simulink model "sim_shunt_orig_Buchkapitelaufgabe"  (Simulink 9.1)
settings: Solver=ode23s  StartTime=0.0  StopTime=4000  RelTol=1e-8  EnableMultiTasking=on
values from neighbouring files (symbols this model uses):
  Bauchdruck = 0    [InitVentil_Buchkapitel.m]
  HydrHoehe = sin(Liegewinkel)*l_Schlauch*73.55    [InitVentil_Buchkapitel.m]
  ICP_n = 0.9330    (= 0.933)    [InitVentil_Buchkapitel.m]
  ICP_shift = 9*sin(Liegewinkel*2 + pi/2)+5 - 14    [InitVentil_Buchkapitel.m]
  R_hyd = 128*eta_Liquor*l_Schlauch/(pi*d_Schlauch^4)*Umrechnungsfaktor    (= 68180382716.6)    [InitVentil_Buchkapitel.m]
  ventil_oeffn = 7    [InitVentil_Buchkapitel.m]
undefined symbols (not defined in the file or in its folder): ABP_n, alph, alphco2, G_vor, h_01, h_02, h_0_ven, ini1_reg, ini2_reg, K_e1, K_e2, K_e_ven, K_G1, K_G2, K_G_ven, k_prod, k_res, K_v1, K_v2, K_v_ven, n_m1, n_m2, O2_verb, p1_n, Pco2_AB, PCO2_soll, Po2_ab, PO2_blut, PO2_soll, r1_100, r2_100, r2_n, r_01, r_02, r_0_ven, r_m1, r_m2, r_t1, r_t2, rv_100, sigma_01, sigma_02, sigma_0_ven, sigma_0_visk_1, sigma_0_visk_2, sigma_koll1, sigma_koll2, sigma_koll_ven, sigma_m01, sigma_m02, V, V1_n, V2_n, V_ven_0, VBPss_n
libraries: neural x36, simulink_extras x3, simulink x1
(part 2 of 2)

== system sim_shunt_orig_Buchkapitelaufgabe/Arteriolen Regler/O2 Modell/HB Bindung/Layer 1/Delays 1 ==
  "p{1}" : Inport  PortDimensions=1
  mux : Mux  Inputs=1
  "pd{1,1}" : Outport
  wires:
  "p{1}"/1 -> mux/1
  mux/1 -> "pd{1,1}"/1

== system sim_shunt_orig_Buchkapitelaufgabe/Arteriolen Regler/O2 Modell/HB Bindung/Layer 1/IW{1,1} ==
  "pd{1,1}" : Inport  PortDimensions=1
  "IW{1,1}(1,:)'" : Constant  Value=-0.064707731186413736
  "IW{1,1}(2,:)'" : Constant  Value=-0.14661098203804576
  Mux : Mux  Inputs=2
  dotprod1 : neural/Weight Functions/dotprod
  dotprod2 : neural/Weight Functions/dotprod
  "iz{1,1}" : Outport
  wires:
  "IW{1,1}(1,:)'"/1 -> dotprod1/1
  dotprod1/1 -> Mux/1
  "IW{1,1}(2,:)'"/1 -> dotprod2/1
  "pd{1,1}"/1 -> dotprod1/2, dotprod2/2
  dotprod2/1 -> Mux/2
  Mux/1 -> "iz{1,1}"/1

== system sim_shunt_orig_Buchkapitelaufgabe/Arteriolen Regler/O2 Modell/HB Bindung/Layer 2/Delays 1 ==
  "p{2}" : Inport  PortDimensions=2
  mux : Mux  Inputs=1
  "pd{2,1}" : Outport
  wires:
  "p{2}"/1 -> mux/1
  mux/1 -> "pd{2,1}"/1

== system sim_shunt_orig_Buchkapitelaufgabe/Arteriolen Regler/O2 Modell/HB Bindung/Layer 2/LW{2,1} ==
  "ad{2,1}" : Inport  PortDimensions=2
  "IW{2,1}(1,:)'" : Constant  Value=[-21.951961087859253;6.8232958826842776]
  Mux : Mux  Inputs=1
  dotprod1 : neural/Weight Functions/dotprod
  "lz{2,1}" : Outport
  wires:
  "IW{2,1}(1,:)'"/1 -> dotprod1/1
  "ad{2,1}"/1 -> dotprod1/2
  dotprod1/1 -> Mux/1
  Mux/1 -> "lz{2,1}"/1

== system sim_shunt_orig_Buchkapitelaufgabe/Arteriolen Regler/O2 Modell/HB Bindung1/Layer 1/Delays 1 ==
  "p{1}" : Inport  PortDimensions=1
  mux : Mux  Inputs=1
  "pd{1,1}" : Outport
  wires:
  mux/1 -> "pd{1,1}"/1
  "p{1}"/1 -> mux/1

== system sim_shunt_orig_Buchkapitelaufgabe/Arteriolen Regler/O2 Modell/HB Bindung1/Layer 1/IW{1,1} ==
  "pd{1,1}" : Inport  PortDimensions=1
  "IW{1,1}(1,:)'" : Constant  Value=-0.064707731186413736
  "IW{1,1}(2,:)'" : Constant  Value=-0.14661098203804576
  Mux : Mux  Inputs=2
  dotprod1 : neural/Weight Functions/dotprod
  dotprod2 : neural/Weight Functions/dotprod
  "iz{1,1}" : Outport
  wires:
  Mux/1 -> "iz{1,1}"/1
  dotprod2/1 -> Mux/2
  "pd{1,1}"/1 -> dotprod2/2, dotprod1/2
  "IW{1,1}(2,:)'"/1 -> dotprod2/1
  dotprod1/1 -> Mux/1
  "IW{1,1}(1,:)'"/1 -> dotprod1/1

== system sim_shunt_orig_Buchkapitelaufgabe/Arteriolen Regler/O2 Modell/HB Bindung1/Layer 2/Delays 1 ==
  "p{2}" : Inport  PortDimensions=2
  mux : Mux  Inputs=1
  "pd{2,1}" : Outport
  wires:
  mux/1 -> "pd{2,1}"/1
  "p{2}"/1 -> mux/1

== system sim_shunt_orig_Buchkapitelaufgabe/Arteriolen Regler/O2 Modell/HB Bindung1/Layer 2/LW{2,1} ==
  "ad{2,1}" : Inport  PortDimensions=2
  "IW{2,1}(1,:)'" : Constant  Value=[-21.951961087859253;6.8232958826842776]
  Mux : Mux  Inputs=1
  dotprod1 : neural/Weight Functions/dotprod
  "lz{2,1}" : Outport
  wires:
  Mux/1 -> "lz{2,1}"/1
  dotprod1/1 -> Mux/1
  "ad{2,1}"/1 -> dotprod1/2
  "IW{2,1}(1,:)'"/1 -> dotprod1/1

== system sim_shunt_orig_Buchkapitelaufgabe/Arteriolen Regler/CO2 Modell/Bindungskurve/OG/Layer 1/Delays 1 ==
  "p{1}" : Inport  PortDimensions=1
  mux : Mux  Inputs=1
  "pd{1,1}" : Outport
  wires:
  mux/1 -> "pd{1,1}"/1
  "p{1}"/1 -> mux/1

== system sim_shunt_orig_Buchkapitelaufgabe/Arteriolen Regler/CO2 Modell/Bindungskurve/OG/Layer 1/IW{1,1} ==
  "pd{1,1}" : Inport  PortDimensions=1
  "IW{1,1}(1,:)'" : Constant  Value=0.39084037748549827
  "IW{1,1}(2,:)'" : Constant  Value=0.022370352278219353
  "IW{1,1}(3,:)'" : Constant  Value=0.19403608090506319
  Mux : Mux  Inputs=3
  dotprod1 : neural/Weight Functions/dotprod
  dotprod2 : neural/Weight Functions/dotprod
  dotprod3 : neural/Weight Functions/dotprod
  "iz{1,1}" : Outport
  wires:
  Mux/1 -> "iz{1,1}"/1
  dotprod3/1 -> Mux/3
  "IW{1,1}(3,:)'"/1 -> dotprod3/1
  dotprod2/1 -> Mux/2
  "pd{1,1}"/1 -> dotprod3/2, dotprod2/2, dotprod1/2
  "IW{1,1}(2,:)'"/1 -> dotprod2/1
  dotprod1/1 -> Mux/1
  "IW{1,1}(1,:)'"/1 -> dotprod1/1

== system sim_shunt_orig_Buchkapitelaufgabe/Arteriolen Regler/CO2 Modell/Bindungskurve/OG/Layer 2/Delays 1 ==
  "p{2}" : Inport  PortDimensions=3
  mux : Mux  Inputs=1
  "pd{2,1}" : Outport
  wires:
  mux/1 -> "pd{2,1}"/1
  "p{2}"/1 -> mux/1

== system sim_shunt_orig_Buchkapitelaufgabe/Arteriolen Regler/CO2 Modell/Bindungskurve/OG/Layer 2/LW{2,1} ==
  "ad{2,1}" : Inport  PortDimensions=3
  "IW{2,1}(1,:)'" : Constant  Value=[-34.807144004972457;79.560951131325595;50.241573431449858]
  Mux : Mux  Inputs=1
  dotprod1 : neural/Weight Functions/dotprod
  "lz{2,1}" : Outport
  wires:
  Mux/1 -> "lz{2,1}"/1
  dotprod1/1 -> Mux/1
  "ad{2,1}"/1 -> dotprod1/2
  "IW{2,1}(1,:)'"/1 -> dotprod1/1

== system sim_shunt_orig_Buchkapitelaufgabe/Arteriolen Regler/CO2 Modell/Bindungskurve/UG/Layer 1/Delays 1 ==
  "p{1}" : Inport  PortDimensions=1
  mux : Mux  Inputs=1
  "pd{1,1}" : Outport
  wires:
  mux/1 -> "pd{1,1}"/1
  "p{1}"/1 -> mux/1

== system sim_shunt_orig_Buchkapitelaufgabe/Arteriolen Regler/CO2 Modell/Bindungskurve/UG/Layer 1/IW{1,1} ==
  "pd{1,1}" : Inport  PortDimensions=1
  "IW{1,1}(1,:)'" : Constant  Value=-0.056170689932274573
  "IW{1,1}(2,:)'" : Constant  Value=0.050617741606017563
  "IW{1,1}(3,:)'" : Constant  Value=0.59403476334946692
  Mux : Mux  Inputs=3
  dotprod1 : neural/Weight Functions/dotprod
  dotprod2 : neural/Weight Functions/dotprod
  dotprod3 : neural/Weight Functions/dotprod
  "iz{1,1}" : Outport
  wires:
  Mux/1 -> "iz{1,1}"/1
  dotprod3/1 -> Mux/3
  "IW{1,1}(3,:)'"/1 -> dotprod3/1
  dotprod2/1 -> Mux/2
  "pd{1,1}"/1 -> dotprod3/2, dotprod2/2, dotprod1/2
  "IW{1,1}(2,:)'"/1 -> dotprod2/1
  dotprod1/1 -> Mux/1
  "IW{1,1}(1,:)'"/1 -> dotprod1/1

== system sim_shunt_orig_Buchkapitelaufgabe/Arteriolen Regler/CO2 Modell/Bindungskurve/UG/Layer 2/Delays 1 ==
  "p{2}" : Inport  PortDimensions=3
  mux : Mux  Inputs=1
  "pd{2,1}" : Outport
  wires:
  mux/1 -> "pd{2,1}"/1
  "p{2}"/1 -> mux/1

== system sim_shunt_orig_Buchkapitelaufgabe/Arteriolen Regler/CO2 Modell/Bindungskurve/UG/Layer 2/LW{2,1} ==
  "ad{2,1}" : Inport  PortDimensions=3
  "IW{2,1}(1,:)'" : Constant  Value=[-73.411517044567987;10.445427355877589;30.151834894692133]
  Mux : Mux  Inputs=1
  dotprod1 : neural/Weight Functions/dotprod
  "lz{2,1}" : Outport
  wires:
  Mux/1 -> "lz{2,1}"/1
  dotprod1/1 -> Mux/1
  "ad{2,1}"/1 -> dotprod1/2
  "IW{2,1}(1,:)'"/1 -> dotprod1/1

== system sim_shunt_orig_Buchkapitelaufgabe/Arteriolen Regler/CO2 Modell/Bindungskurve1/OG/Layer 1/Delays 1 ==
  "p{1}" : Inport  PortDimensions=1
  mux : Mux  Inputs=1
  "pd{1,1}" : Outport
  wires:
  "p{1}"/1 -> mux/1
  mux/1 -> "pd{1,1}"/1

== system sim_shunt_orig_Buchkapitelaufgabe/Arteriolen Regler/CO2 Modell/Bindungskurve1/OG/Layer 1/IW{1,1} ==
  "pd{1,1}" : Inport  PortDimensions=1
  "IW{1,1}(1,:)'" : Constant  Value=0.39084037748549827
  "IW{1,1}(2,:)'" : Constant  Value=0.022370352278219353
  "IW{1,1}(3,:)'" : Constant  Value=0.19403608090506319
  Mux : Mux  Inputs=3
  dotprod1 : neural/Weight Functions/dotprod
  dotprod2 : neural/Weight Functions/dotprod
  dotprod3 : neural/Weight Functions/dotprod
  "iz{1,1}" : Outport
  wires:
  "IW{1,1}(1,:)'"/1 -> dotprod1/1
  dotprod1/1 -> Mux/1
  "IW{1,1}(2,:)'"/1 -> dotprod2/1
  "pd{1,1}"/1 -> dotprod1/2, dotprod2/2, dotprod3/2
  dotprod2/1 -> Mux/2
  "IW{1,1}(3,:)'"/1 -> dotprod3/1
  dotprod3/1 -> Mux/3
  Mux/1 -> "iz{1,1}"/1

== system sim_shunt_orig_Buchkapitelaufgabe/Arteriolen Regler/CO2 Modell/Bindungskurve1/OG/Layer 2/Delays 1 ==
  "p{2}" : Inport  PortDimensions=3
  mux : Mux  Inputs=1
  "pd{2,1}" : Outport
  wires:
  "p{2}"/1 -> mux/1
  mux/1 -> "pd{2,1}"/1

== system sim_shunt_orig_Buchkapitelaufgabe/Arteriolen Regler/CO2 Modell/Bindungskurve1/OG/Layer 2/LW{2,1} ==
  "ad{2,1}" : Inport  PortDimensions=3
  "IW{2,1}(1,:)'" : Constant  Value=[-34.807144004972457;79.560951131325595;50.241573431449858]
  Mux : Mux  Inputs=1
  dotprod1 : neural/Weight Functions/dotprod
  "lz{2,1}" : Outport
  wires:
  "IW{2,1}(1,:)'"/1 -> dotprod1/1
  "ad{2,1}"/1 -> dotprod1/2
  dotprod1/1 -> Mux/1
  Mux/1 -> "lz{2,1}"/1

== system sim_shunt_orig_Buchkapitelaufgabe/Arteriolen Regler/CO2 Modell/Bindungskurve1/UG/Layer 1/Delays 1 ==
  "p{1}" : Inport  PortDimensions=1
  mux : Mux  Inputs=1
  "pd{1,1}" : Outport
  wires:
  "p{1}"/1 -> mux/1
  mux/1 -> "pd{1,1}"/1

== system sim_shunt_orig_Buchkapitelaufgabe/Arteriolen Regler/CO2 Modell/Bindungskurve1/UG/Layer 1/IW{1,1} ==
  "pd{1,1}" : Inport  PortDimensions=1
  "IW{1,1}(1,:)'" : Constant  Value=-0.056170689932274573
  "IW{1,1}(2,:)'" : Constant  Value=0.050617741606017563
  "IW{1,1}(3,:)'" : Constant  Value=0.59403476334946692
  Mux : Mux  Inputs=3
  dotprod1 : neural/Weight Functions/dotprod
  dotprod2 : neural/Weight Functions/dotprod
  dotprod3 : neural/Weight Functions/dotprod
  "iz{1,1}" : Outport
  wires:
  "IW{1,1}(1,:)'"/1 -> dotprod1/1
  dotprod1/1 -> Mux/1
  "IW{1,1}(2,:)'"/1 -> dotprod2/1
  "pd{1,1}"/1 -> dotprod1/2, dotprod2/2, dotprod3/2
  dotprod2/1 -> Mux/2
  "IW{1,1}(3,:)'"/1 -> dotprod3/1
  dotprod3/1 -> Mux/3
  Mux/1 -> "iz{1,1}"/1

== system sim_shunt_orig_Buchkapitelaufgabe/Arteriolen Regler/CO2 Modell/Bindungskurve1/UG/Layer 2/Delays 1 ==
  "p{2}" : Inport  PortDimensions=3
  mux : Mux  Inputs=1
  "pd{2,1}" : Outport
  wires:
  "p{2}"/1 -> mux/1
  mux/1 -> "pd{2,1}"/1

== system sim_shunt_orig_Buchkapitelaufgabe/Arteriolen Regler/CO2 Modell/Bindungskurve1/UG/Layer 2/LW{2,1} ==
  "ad{2,1}" : Inport  PortDimensions=3
  "IW{2,1}(1,:)'" : Constant  Value=[-73.411517044567987;10.445427355877589;30.151834894692133]
  Mux : Mux  Inputs=1
  dotprod1 : neural/Weight Functions/dotprod
  "lz{2,1}" : Outport
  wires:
  "IW{2,1}(1,:)'"/1 -> dotprod1/1
  "ad{2,1}"/1 -> dotprod1/2
  dotprod1/1 -> Mux/1
  Mux/1 -> "lz{2,1}"/1
